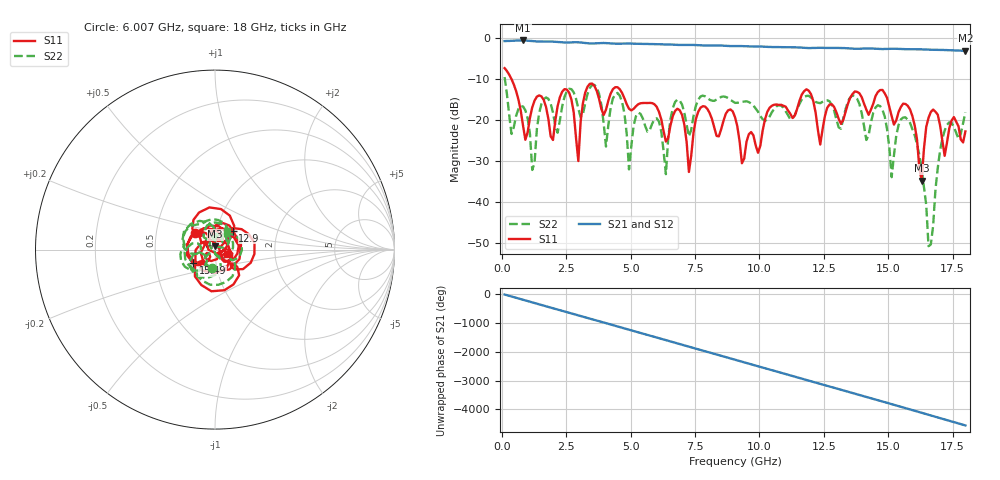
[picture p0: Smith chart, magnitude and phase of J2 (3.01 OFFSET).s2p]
!Agilent Technologies,E8364B,MY43040528,A.07.50.67
!Agilent E8364B: A.07.50.67
!Date: Wednesday, May 04, 2022 12:40:19
!Correction: S11(Full 2 Port(1,2))
!S21(Full 2 Port(1,2))
!S12(Full 2 Port(1,2))
!S22(Full 2 Port(1,2))
!S2P File: Measurements: S11, S21, S12, S22:
# Hz S  dB  R 50
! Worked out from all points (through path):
!   201 points, 100 MHz to 18 GHz, reference 50 ohm
!   highest |S21| = -0.58 dB at 816 MHz (marker M1); lowest = -3.1 dB at 18 GHz (marker M2)
!   group delay of S21, straight-line fit = 701 ps
!   lowest |S11| = -34.8 dB at 16.3 GHz (marker M3), VSWR 1.04, Z = 50.1 + j1.81 ohm
!   |S11| at or under -10 dB: 367 MHz to end of sweep
!   |S22| runs from -50.8 to -9.5 dB; largest |S21 - S12| = 0.013
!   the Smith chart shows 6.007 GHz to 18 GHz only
!   S11 on the Smith chart (normalised r, x): 6.007 GHz: 0.79, +0.15; 12.9 GHz: 1.19, +0.26; 15.49 GHz: 0.77, -0.12; 18 GHz: 1.15, -0.05
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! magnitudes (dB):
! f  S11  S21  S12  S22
! 100 MHz  -7.3  -0.7  -0.7  -9.5
! 816 MHz  -21.4  -0.6  -0.5  -16.7
! 1.174 GHz  -16.9  -0.7  -0.7  -32.2
! 1.621 GHz  -15.1  -0.9  -0.8  -14.9
! 2.606 GHz  -13.3  -1.1  -1.0  -12.4
! 2.964 GHz  -30.0  -1.0  -1.0  -17.2
! 3.143 GHz  -15.9  -1.1  -1.1  -18.5
! 4.486 GHz  -12.0  -1.4  -1.3  -13.4
! 4.933 GHz  -17.2  -1.3  -1.3  -32.0
! 6.007 GHz  -16.8  -1.5  -1.4  -19.6
! 6.096 GHz  -18.0  -1.5  -1.4  -20.4
! 7.26 GHz  -32.7  -1.7  -1.6  -24.0
! 7.707 GHz  -17.0  -1.8  -1.7  -14.3
! 9.05 GHz  -19.3  -1.9  -1.9  -15.8
! 12.09 GHz  -15.4  -2.4  -2.3  -14.9
! 12.9 GHz  -16.8  -2.4  -2.3  -17.6
! 15.05 GHz  -16.9  -2.6  -2.6  -26.8
! 15.49 GHz  -16.8  -2.7  -2.6  -19.9
! 16.3 GHz  -34.8  -2.7  -2.7  -31.9
! 16.66 GHz  -18.0  -2.8  -2.8  -50.4
! 17.11 GHz  -24.9  -2.9  -2.8  -24.5
! 18 GHz  -22.8  -3.1  -3.0  -18.1
